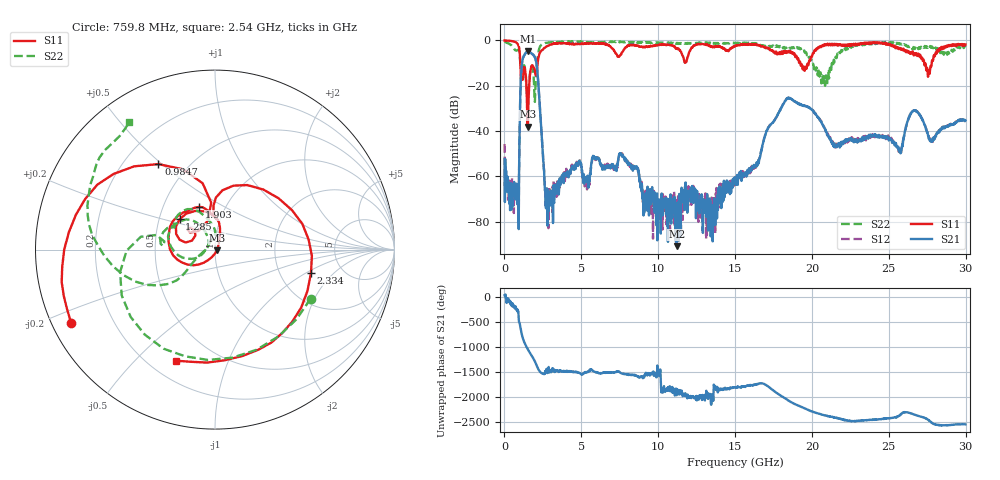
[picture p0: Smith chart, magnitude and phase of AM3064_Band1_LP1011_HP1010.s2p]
# Hz S DB R 50.0
!freq dBS11 angS11 dBS21 angS21 dBS12 angS12 dBS22 angS22
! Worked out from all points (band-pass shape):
!   1600 points, 10 MHz to 29.98 GHz, reference 50 ohm
!   highest |S21| = -4.89 dB at 1.528 GHz (marker M1); lowest = -90.9 dB at 11.2 GHz (marker M2)
!   |S21| within 3 dB of the highest: 1.203 GHz to 2.002 GHz (799.5 MHz wide, 49.9 % of centre)
!   lowest |S11| = -38.1 dB at 1.51 GHz (marker M3), VSWR 1.03, Z = 51.2 - j0.426 ohm
!   |S11| at or under -10 dB: 1.031 GHz to 2.158 GHz (1.127 GHz wide, 70.7 % of centre); 19.25 GHz to 19.79 GHz (545.7 MHz wide, 2.8 % of centre); 27.3 GHz to 27.79 GHz (486.6 MHz wide, 1.77 % of centre)
!   |S22| runs from -27.2 to -0.3 dB; largest |S21 - S12| = 0.0087
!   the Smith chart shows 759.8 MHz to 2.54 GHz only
!   S11 on the Smith chart (normalised r, x): 759.8 MHz: 0.06, -0.24; 984.7 MHz: 0.34, +0.49; 1.285 GHz: 0.64, +0.23; 1.903 GHz: 0.75, +0.38; 2.334 GHz: 2.99, -1.11; 2.54 GHz: 0.31, -0.67
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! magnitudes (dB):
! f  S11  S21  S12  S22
! 10 MHz  0.0  -52.4  -45.8  -0.3
! 759.8 MHz  -0.9  -67.7  -64.1  -4.5
! 984.7 MHz  -4.9  -40.6  -40.7  -6.2
! 1.285 GHz  -11.7  -6.6  -6.6  -11.0
! 1.51 GHz  -38.1  -4.9  -4.9  -26.9
! 1.528 GHz  -36.5  -4.9  -4.9  -25.3
! 1.903 GHz  -11.9  -6.6  -6.6  -16.5
! 2.334 GHz  -5.2  -32.7  -32.7  -2.5
! 2.54 GHz  -3.7  -53.7  -54.6  -1.4
! 2.822 GHz  -2.3  -66.1  -70.2  -1.0
! 5.015 GHz  -1.4  -56.1  -55.9  -0.7
! 7.62 GHz  -5.7  -50.3  -49.8  -0.7
! 10 GHz  -2.0  -72.4  -72.9  -1.0
! 11.2 GHz  -3.6  -90.9  -73.4  -1.2
! 15 GHz  -2.5  -61.5  -63.0  -1.3
! 18.34 GHz  -5.5  -26.0  -25.8  -3.4
! 19.99 GHz  -7.2  -30.7  -30.6  -9.2
! 21.51 GHz  -1.6  -46.5  -46.0  -8.6
! 25 GHz  -1.4  -44.2  -42.7  -1.1
! 26.66 GHz  -5.7  -30.9  -30.9  -3.6
! 27.56 GHz  -15.8  -42.3  -42.4  -2.6
! 29.98 GHz  -1.8  -35.4  -35.3  -3.0
